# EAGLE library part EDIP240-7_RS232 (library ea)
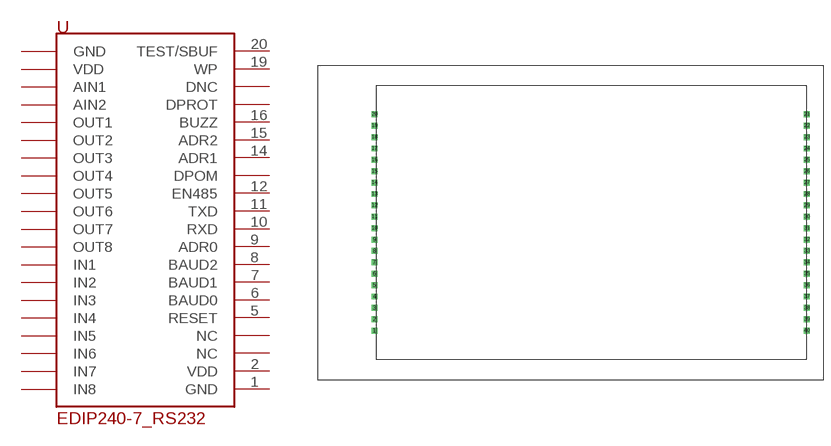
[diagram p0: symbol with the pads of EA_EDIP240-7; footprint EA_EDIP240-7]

Designator prefix -

## EDIP240-7_RS232  [EA_EDIP240-7]
1  GND  pwr
2  VDD  pwr
5  RESET  in
6  BAUD0  in
7  BAUD1  in
8  BAUD2  in
9  ADR0  in
10  RXD  in
11  TXD  out
12  EN485  out
14  ADR1  in
15  ADR2  in
16  BUZZ  out
19  WP  in
20  TEST/SBUF

## Footprint EA_EDIP240-7 (pad centres in mm)
drill 0.813 square: 1 0,0; 2 0,2.54; 3 0,5.08; 4 0,7.62; 5 0,10.16; 6 0,12.7; 7 0,15.24; 8 0,17.78; 9 0,20.32; 10 0,22.86; 11 0,25.4; 12 0,27.94; 13 0,30.48; 14 0,33.02; 15 0,35.56; 16 0,38.1; 17 0,40.64; 18 0,43.18; 19 0,45.72; 20 0,48.26; 21 96.52,48.26; 22 96.52,45.72; 23 96.52,43.18; 24 96.52,40.64; 25 96.52,38.1; 26 96.52,35.56; 27 96.52,33.02; 28 96.52,30.48; 29 96.52,27.94; 30 96.52,25.4; 31 96.52,22.86; 32 96.52,20.32; 33 96.52,17.78; 34 96.52,15.24; 35 96.52,12.7; 36 96.52,10.16; 37 96.52,7.62; 38 96.52,5.08; 39 96.52,2.54; 40 96.52,0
